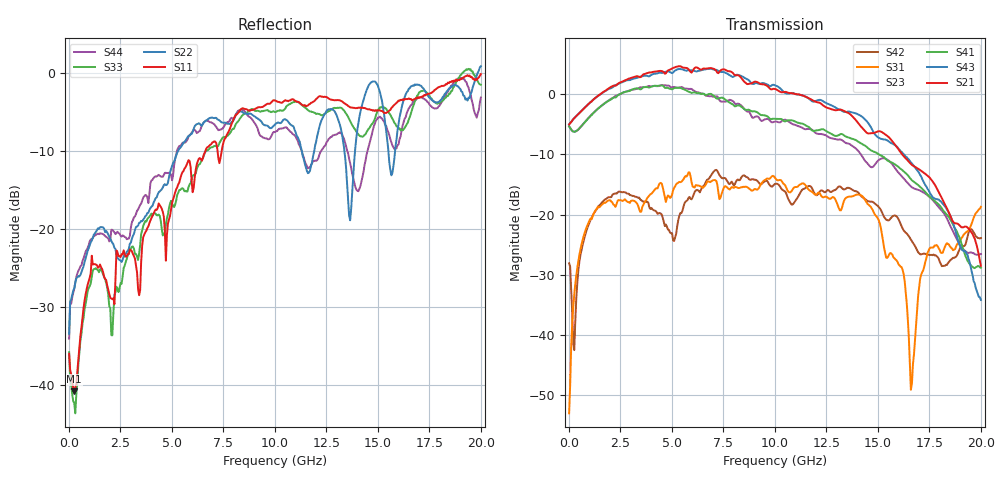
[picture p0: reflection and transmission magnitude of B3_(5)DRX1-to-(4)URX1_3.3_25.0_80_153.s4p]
!Agilent Technologies,N5225A,MY51451112,A.09.50.13
!Agilent N5225A: A.09.50.13
!Date: Sunday, March 12, 2017 05:22:19
!Correction: S11(Full 4 Port(1,2,3,4))
!S12(Full 4 Port(1,2,3,4))
!S13(Full 4 Port(1,2,3,4))
!S14(Full 4 Port(1,2,3,4))
!S21(Full 4 Port(1,2,3,4))
!S22(Full 4 Port(1,2,3,4))
!S23(Full 4 Port(1,2,3,4))
!S24(Full 4 Port(1,2,3,4))
!S31(Full 4 Port(1,2,3,4))
!S32(Full 4 Port(1,2,3,4))
!S33(Full 4 Port(1,2,3,4))
!S34(Full 4 Port(1,2,3,4))
!S41(Full 4 Port(1,2,3,4))
!S42(Full 4 Port(1,2,3,4))
!S43(Full 4 Port(1,2,3,4))
!S44(Full 4 Port(1,2,3,4))
!S4P File: Measurements: <S11,S12,S13,S14>,
!<S21,S22,S23,S24>,
!<S31,S32,S33,S34>,
!<S41,S42,S43,S44>:
# Hz S  dB  R 50
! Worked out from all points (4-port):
!   401 points, 10 MHz to 20 GHz, reference 50 ohm
!   strongest paths, dB at 10 MHz, 5.008 GHz, 10.01 GHz, 15 GHz, 20 GHz:
!     S21: -5.0, 4.3, 0.9, -6.2, -28.5
!     S43: -5.0, 3.5, 1.5, -7.1, -34.2
!     S41: -5.3, 0.8, -4.1, -9.9, -28.8
!     S23: -5.3, 1.1, -4.5, -11.1, -26.5
!     S31: -53.0, -16.7, -13.9, -20.6, -18.7
!     S42: -28.1, -23.1, -14.9, -18.6, -23.9
!   lowest |S11| = -40.9 dB at 259.9 MHz (marker M1), VSWR 1.02, Z = 50.3 - j0.868 ohm
!   |S11| at or under -10 dB: start of sweep to 6.63 GHz; 7.214 GHz to 7.418 GHz (204.1 MHz wide, 2.79 % of centre)
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1e7  -36.01 -39.1  -64.72 138.0  -53.59 19.9  -63.25 138.5
     -5.02 1.7  -33.45 39.4  -5.33 -179.7  -27.95 37.9
     -52.98 16.9  -69.93 130.7  -35.82 -46.2  -62.26 140.9
     -5.33 -179.7  -28.07 38.1  -5.00 1.8  -34.08 43.9
2.59875e8  -40.85 -72.3  -49.57 56.6  -33.07 94.9  -50.37 52.9
           -3.97 2.2  -27.62 -131.9  -6.23 175.5  -41.87 -161.6
           -33.25 95.2  -49.60 57.3  -42.35 -79.2  -50.31 56.4
           -6.23 174.7  -42.49 -170.5  -3.95 1.5  -27.68 -137.8
3.058475e9  -22.88 139.2  -43.22 -16.8  -17.63 50.4  -42.83 -24.3
            2.75 -97.5  -21.26 160.8  0.73 72.8  -16.92 38.1
            -17.65 51.5  -41.49 -12.0  -22.30 114.0  -41.29 -21.3
            0.76 63.4  -16.86 38.2  2.49 -104.9  -19.16 139.9
5.10745e9  -15.84 88.9  -38.97 9.7  -15.74 28.0  -38.78 -27.6
           4.43 170.4  -11.39 145.1  1.21 -26.8  -24.61 49.2
           -15.54 27.1  -37.55 -3.2  -17.21 104.0  -35.61 -52.5
           1.02 -41.9  -24.36 52.3  3.79 160.5  -11.85 126.8
8.255875e9  -5.01 36.3  -39.84 -109.6  -15.79 1.4  -36.40 -138.9
            3.10 13.8  -5.02 80.8  -1.62 -172.7  -13.89 46.9
            -15.58 0.2  -32.45 -115.9  -6.07 58.1  -31.75 -152.2
            -1.83 164.2  -14.29 50.6  3.17 1.1  -4.83 45.8
1.16042e10  -4.19 -7.3  -37.34 -117.7  -15.23 -23.3  -39.31 -132.4
            -0.58 -130.3  -12.88 81.1  -5.76 46.3  -15.45 36.8
            -15.70 -23.6  -34.10 -127.5  -4.78 10.2  -33.81 -155.1
            -5.37 7.7  -15.28 41.2  -0.61 -155.8  -12.24 23.0
2e10  -0.18 -114.1  -33.02 62.6  -18.73 121.3  -35.48 21.4
      -28.48 -157.8  0.84 17.1  -26.52 24.9  -23.90 102.0
      -18.70 121.4  -34.04 40.8  -1.54 -87.7  -35.23 -7.6
      -28.83 -21.5  -23.88 102.7  -34.15 174.5  -3.18 -136.6
